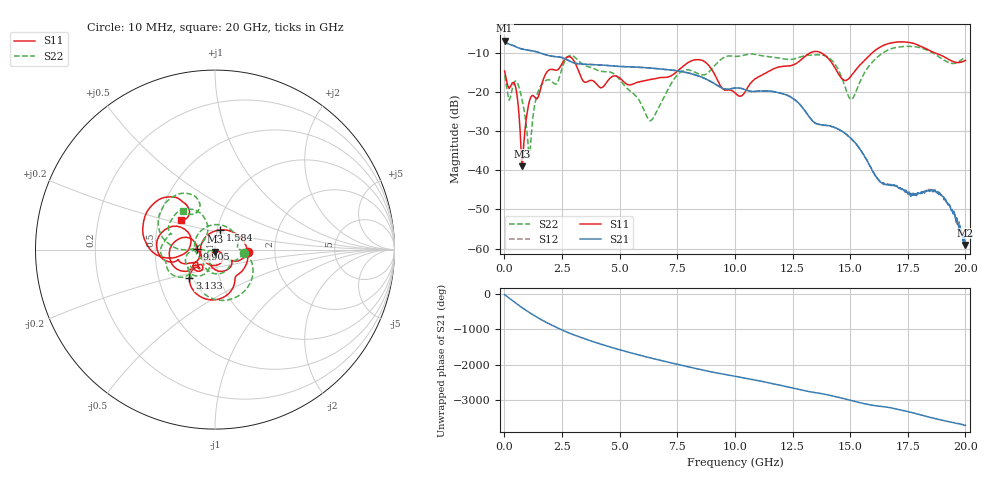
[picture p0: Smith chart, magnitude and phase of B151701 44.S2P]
!  2-Port S-parameters saved by WinCal
! VAR MeasName=S-Parameters (CALIBRATED_DATA) read from VNA (N5244A)
! VAR MeasDate=2015-12-24 19:14:37
! VAR NAME=B151701 44
! VAR FILENAME=B151701 44.S2P
! VAR DATE=2015-12-24 19:14:37
! VAR PHYS_PORTS=1,3
# Hz S DB R 50
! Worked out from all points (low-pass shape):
!   801 points, 10 MHz to 20 GHz, reference 50 ohm
!   highest |S21| = -6.94 dB at 10 MHz (marker M1); lowest = -59.1 dB at 20 GHz (marker M2)
!   |S21| within 3 dB of the highest: start of sweep to 1.462 GHz
!   lowest |S11| = -39.0 dB at 759.6 MHz (marker M3), VSWR 1.02, Z = 50 - j1.12 ohm
!   |S11| at or under -10 dB: start of sweep to 13.3 GHz; 13.71 GHz to 15.98 GHz (2.267 GHz wide, 15.3 % of centre); 18.64 GHz to end of sweep
!   |S22| runs from -36.6 to -8.4 dB; largest |S21 - S12| = 0.0013
!   S11 on the Smith chart (normalised r, x): 10 MHz: 1.45, -0.05; 1.584 GHz: 1.03, +0.23; 3.133 GHz: 0.72, -0.24; 9.905 GHz: 0.81, +0.00; 20 GHz: 0.65, +0.22
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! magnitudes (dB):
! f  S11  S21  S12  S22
! 10 MHz  -14.7  -6.9  -6.9  -15.9
! 209.9 MHz  -19.2  -7.9  -7.9  -22.2
! 484.8 MHz  -18.8  -8.5  -8.5  -17.3
! 759.6 MHz  -39.0  -9.1  -9.1  -21.9
! 1.084 GHz  -22.4  -9.5  -9.4  -36.6
! 1.584 GHz  -19.0  -10.2  -10.2  -18.5
! 3.133 GHz  -13.5  -12.8  -12.8  -11.6
! 3.358 GHz  -16.7  -13.0  -13.0  -12.9
! 4.808 GHz  -16.0  -13.5  -13.5  -15.7
! 6.307 GHz  -16.9  -14.0  -13.9  -27.4
! 6.682 GHz  -16.5  -14.2  -14.1  -24.1
! 7.606 GHz  -14.3  -14.8  -14.8  -15.2
! 8.481 GHz  -11.8  -16.1  -16.1  -15.6
! 9.905 GHz  -19.8  -19.2  -19.2  -10.9
! 10.01 GHz  -20.3  -19.1  -19.0  -11.0
! 12.3 GHz  -13.4  -21.0  -21.0  -11.8
! 13.35 GHz  -9.9  -27.3  -27.3  -10.7
! 14.25 GHz  -13.0  -29.0  -28.9  -12.3
! 15.05 GHz  -15.9  -32.0  -32.1  -21.9
! 16.68 GHz  -7.7  -43.7  -43.7  -9.3
! 18.98 GHz  -10.8  -46.6  -46.4  -11.6
! 20 GHz  -12.0  -59.1  -59.0  -11.1
